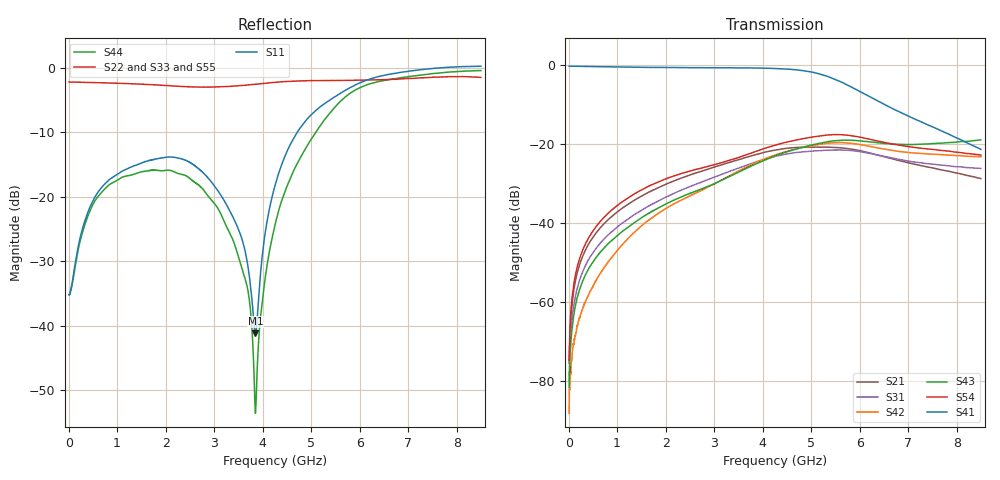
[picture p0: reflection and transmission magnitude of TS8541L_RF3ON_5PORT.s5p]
! Created with skrf (http://scikit-rf.org).
# Hz S RI R 50.0
!freq ReS11 ImS11 ReS12 ImS12 ReS13 ImS13
! ReS14 ImS14 ReS15 ImS15
! ReS21 ImS21 ReS22 ImS22 ReS23 ImS23
! ReS24 ImS24 ReS25 ImS25
! ReS31 ImS31 ReS32 ImS32 ReS33 ImS33
! ReS34 ImS34 ReS35 ImS35
! ReS41 ImS41 ReS42 ImS42 ReS43 ImS43
! ReS44 ImS44 ReS45 ImS45
! ReS51 ImS51 ReS52 ImS52 ReS53 ImS53
! ReS54 ImS54 ReS55 ImS55
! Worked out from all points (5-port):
!   1601 points, 10 MHz to 8.5 GHz, reference 50 ohm
!   strongest paths, dB at 10 MHz, 2.132 GHz, 4.255 GHz, 6.378 GHz, 8.5 GHz:
!     S41: -0.2, -0.5, -0.8, -9.0, -21.3
!     S54: -74.8, -28.2, -20.2, -19.2, -22.7
!     S43: -81.7, -34.4, -22.9, -19.6, -18.9
!     S42: -88.2, -35.4, -22.7, -20.9, -23.1
!     S31: -79.9, -32.7, -23.1, -22.7, -26.1
!     S21: -75.5, -29.5, -21.5, -22.7, -28.7
!   lowest |S11| = -41.2 dB at 3.852 GHz (marker M1), VSWR 1.02, Z = 49.1 + j0.119 ohm
!   |S11| at or under -10 dB: start of sweep to 4.715 GHz
